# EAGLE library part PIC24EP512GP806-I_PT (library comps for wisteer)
PIC24EP512GP806-I/PT: Pic with 512KB rom, 50KB ram, 60/70Mhz, 64 pins http://ww1.microchip.com/downloads/en/DeviceDoc/70616g.pdf
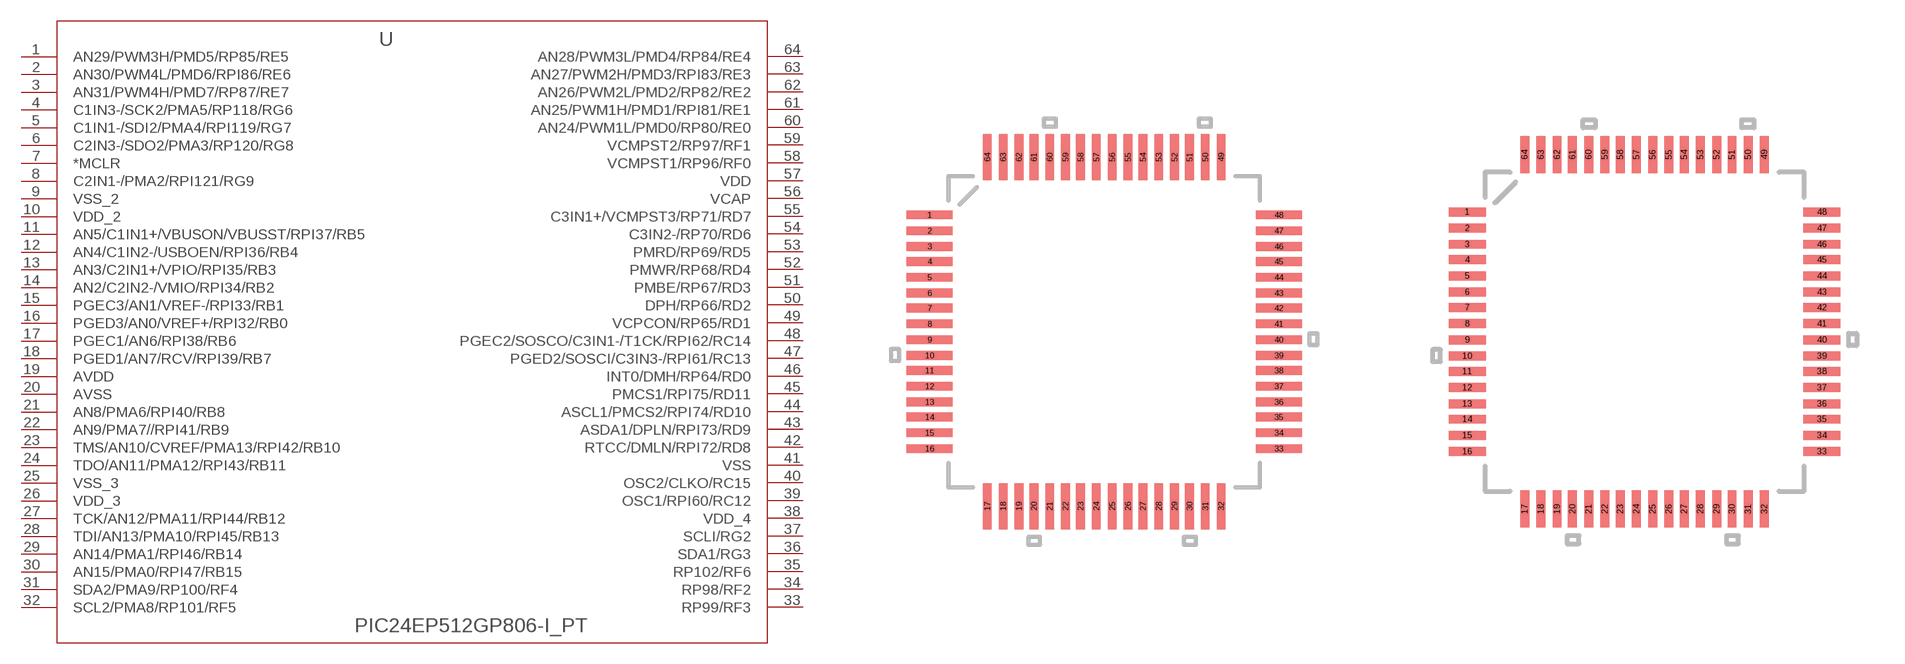
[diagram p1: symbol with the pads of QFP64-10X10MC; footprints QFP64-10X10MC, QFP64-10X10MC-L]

Designator prefix U

## PIC24EP512GP806-I_PT (MANUFACTURER_PART_NUMBER: dspic33ep256mu806-x_pt; VENDOR: MICROCHIP)  [QFP64-10X10MC]
1  AN29/PWM3H/PMD5/RP85/RE5  pas
2  AN30/PWM4L/PMD6/RPI86/RE6  pas
3  AN31/PWM4H/PMD7/RP87/RE7  pas
4  C1IN3-/SCK2/PMA5/RP118/RG6  pas
5  C1IN1-/SDI2/PMA4/RPI119/RG7  pas
6  C2IN3-/SDO2/PMA3/RP120/RG8  pas
7  *MCLR  in
8  C2IN1-/PMA2/RPI121/RG9  pas
9  VSS_2  pwr
10  VDD_2  pwr
11  AN5/C1IN1+/VBUSON/VBUSST/RPI37/RB5  pas
12  AN4/C1IN2-/USBOEN/RPI36/RB4  pas
13  AN3/C2IN1+/VPIO/RPI35/RB3  pas
14  AN2/C2IN2-/VMIO/RPI34/RB2  pas
15  PGEC3/AN1/VREF-/RPI33/RB1  pas
16  PGED3/AN0/VREF+/RPI32/RB0  pas
17  PGEC1/AN6/RPI38/RB6  pas
18  PGED1/AN7/RCV/RPI39/RB7  pas
19  AVDD  pwr
20  AVSS  pwr
21  AN8/PMA6/RPI40/RB8  pas
22  AN9/PMA7//RPI41/RB9  pas
23  TMS/AN10/CVREF/PMA13/RPI42/RB10  pas
24  TDO/AN11/PMA12/RPI43/RB11  pas
25  VSS_3  pwr
26  VDD_3  pwr
27  TCK/AN12/PMA11/RPI44/RB12  pas
28  TDI/AN13/PMA10/RPI45/RB13  pas
29  AN14/PMA1/RPI46/RB14  pas
30  AN15/PMA0/RPI47/RB15  pas
31  SDA2/PMA9/RP100/RF4  pas
32  SCL2/PMA8/RP101/RF5  pas
33  RP99/RF3  pas
34  RP98/RF2  pwr
35  RP102/RF6  pwr
36  SDA1/RG3  pas
37  SCLI/RG2  pas
38  VDD_4  pwr
39  OSC1/RPI60/RC12  pas
40  OSC2/CLKO/RC15  pas
41  VSS  pwr
42  RTCC/DMLN/RPI72/RD8  pas
43  ASDA1/DPLN/RPI73/RD9  pas
44  ASCL1/PMCS2/RPI74/RD10  pas
45  PMCS1/RPI75/RD11  pas
46  INT0/DMH/RP64/RD0  pas
47  PGED2/SOSCI/C3IN3-/RPI61/RC13  pas
48  PGEC2/SOSCO/C3IN1-/T1CK/RPI62/RC14  pas
49  VCPCON/RP65/RD1  pas
50  DPH/RP66/RD2  pas
51  PMBE/RP67/RD3  pas
52  PMWR/RP68/RD4  pas
53  PMRD/RP69/RD5  pas
54  C3IN2-/RP70/RD6  pas
55  C3IN1+/VCMPST3/RP71/RD7  pas
56  VCAP  pwr
57  VDD  pwr
58  VCMPST1/RP96/RF0  pas
59  VCMPST2/RP97/RF1  pas
60  AN24/PWM1L/PMD0/RP80/RE0  pas
61  AN25/PWM1H/PMD1/RPI81/RE1  pas
62  AN26/PWM2L/PMD2/RP82/RE2  pas
63  AN27/PWM2H/PMD3/RPI83/RE3  pas
64  AN28/PWM3L/PMD4/RP84/RE4  pas

## PIC24EP512GP806-I_PTL  [QFP64-10X10MC-L]
Pads as for QFP64-10X10MC

## PIC24EP512GP806-I_PTM  [QFP64-10X10MC-M]
Pads as for QFP64-10X10MC

## Footprint QFP64-10X10MC (pad centres in mm)
smd 1.473 x 0.279: 1 -5.613,3.759; 2 -5.613,3.251; 3 -5.613,2.743; 4 -5.613,2.261; 5 -5.613,1.753; 6 -5.613,1.245; 7 -5.613,0.762; 8 -5.613,0.254; 9 -5.613,-0.254; 10 -5.613,-0.762; 11 -5.613,-1.245; 12 -5.613,-1.753; 13 -5.613,-2.261; 14 -5.613,-2.743; 15 -5.613,-3.251; 16 -5.613,-3.759; 33 5.613,-3.759; 34 5.613,-3.251; 35 5.613,-2.743; 36 5.613,-2.261; 37 5.613,-1.753; 38 5.613,-1.245; 39 5.613,-0.762; 40 5.613,-0.254; 41 5.613,0.254; 42 5.613,0.762; 43 5.613,1.245; 44 5.613,1.753; 45 5.613,2.261; 46 5.613,2.743; 47 5.613,3.251; 48 5.613,3.759
smd 0.279 x 1.473: 17 -3.759,-5.613; 18 -3.251,-5.613; 19 -2.743,-5.613; 20 -2.261,-5.613; 21 -1.753,-5.613; 22 -1.245,-5.613; 23 -0.762,-5.613; 24 -0.254,-5.613; 25 0.254,-5.613; 26 0.762,-5.613; 27 1.245,-5.613; 28 1.753,-5.613; 29 2.261,-5.613; 30 2.743,-5.613; 31 3.251,-5.613; 32 3.759,-5.613; 49 3.759,5.613; 50 3.251,5.613; 51 2.743,5.613; 52 2.261,5.613; 53 1.753,5.613; 54 1.245,5.613; 55 0.762,5.613; 56 0.254,5.613; 57 -0.254,5.613; 58 -0.762,5.613; 59 -1.245,5.613; 60 -1.753,5.613; 61 -2.261,5.613; 62 -2.743,5.613; 63 -3.251,5.613; 64 -3.759,5.613

## Footprint QFP64-10X10MC-L (pad centres in mm)
smd 1.168 x 0.279: 1 -5.563,3.759; 2 -5.563,3.251; 3 -5.563,2.743; 4 -5.563,2.261; 5 -5.563,1.753; 6 -5.563,1.245; 7 -5.563,0.762; 8 -5.563,0.254; 9 -5.563,-0.254; 10 -5.563,-0.762; 11 -5.563,-1.245; 12 -5.563,-1.753; 13 -5.563,-2.261; 14 -5.563,-2.743; 15 -5.563,-3.251; 16 -5.563,-3.759; 33 5.563,-3.759; 34 5.563,-3.251; 35 5.563,-2.743; 36 5.563,-2.261; 37 5.563,-1.753; 38 5.563,-1.245; 39 5.563,-0.762; 40 5.563,-0.254; 41 5.563,0.254; 42 5.563,0.762; 43 5.563,1.245; 44 5.563,1.753; 45 5.563,2.261; 46 5.563,2.743; 47 5.563,3.251; 48 5.563,3.759
smd 0.279 x 1.168: 17 -3.759,-5.563; 18 -3.251,-5.563; 19 -2.743,-5.563; 20 -2.261,-5.563; 21 -1.753,-5.563; 22 -1.245,-5.563; 23 -0.762,-5.563; 24 -0.254,-5.563; 25 0.254,-5.563; 26 0.762,-5.563; 27 1.245,-5.563; 28 1.753,-5.563; 29 2.261,-5.563; 30 2.743,-5.563; 31 3.251,-5.563; 32 3.759,-5.563; 49 3.759,5.563; 50 3.251,5.563; 51 2.743,5.563; 52 2.261,5.563; 53 1.753,5.563; 54 1.245,5.563; 55 0.762,5.563; 56 0.254,5.563; 57 -0.254,5.563; 58 -0.762,5.563; 59 -1.245,5.563; 60 -1.753,5.563; 61 -2.261,5.563; 62 -2.743,5.563; 63 -3.251,5.563; 64 -3.759,5.563

## Footprint QFP64-10X10MC-M (pad centres in mm)
smd 1.778 x 0.279: 1 -5.664,3.759; 2 -5.664,3.251; 3 -5.664,2.743; 4 -5.664,2.261; 5 -5.664,1.753; 6 -5.664,1.245; 7 -5.664,0.762; 8 -5.664,0.254; 9 -5.664,-0.254; 10 -5.664,-0.762; 11 -5.664,-1.245; 12 -5.664,-1.753; 13 -5.664,-2.261; 14 -5.664,-2.743; 15 -5.664,-3.251; 16 -5.664,-3.759; 33 5.664,-3.759; 34 5.664,-3.251; 35 5.664,-2.743; 36 5.664,-2.261; 37 5.664,-1.753; 38 5.664,-1.245; 39 5.664,-0.762; 40 5.664,-0.254; 41 5.664,0.254; 42 5.664,0.762; 43 5.664,1.245; 44 5.664,1.753; 45 5.664,2.261; 46 5.664,2.743; 47 5.664,3.251; 48 5.664,3.759
smd 0.279 x 1.778: 17 -3.759,-5.664; 18 -3.251,-5.664; 19 -2.743,-5.664; 20 -2.261,-5.664; 21 -1.753,-5.664; 22 -1.245,-5.664; 23 -0.762,-5.664; 24 -0.254,-5.664; 25 0.254,-5.664; 26 0.762,-5.664; 27 1.245,-5.664; 28 1.753,-5.664; 29 2.261,-5.664; 30 2.743,-5.664; 31 3.251,-5.664; 32 3.759,-5.664; 49 3.759,5.664; 50 3.251,5.664; 51 2.743,5.664; 52 2.261,5.664; 53 1.753,5.664; 54 1.245,5.664; 55 0.762,5.664; 56 0.254,5.664; 57 -0.254,5.664; 58 -0.762,5.664; 59 -1.245,5.664; 60 -1.753,5.664; 61 -2.261,5.664; 62 -2.743,5.664; 63 -3.251,5.664; 64 -3.759,5.664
